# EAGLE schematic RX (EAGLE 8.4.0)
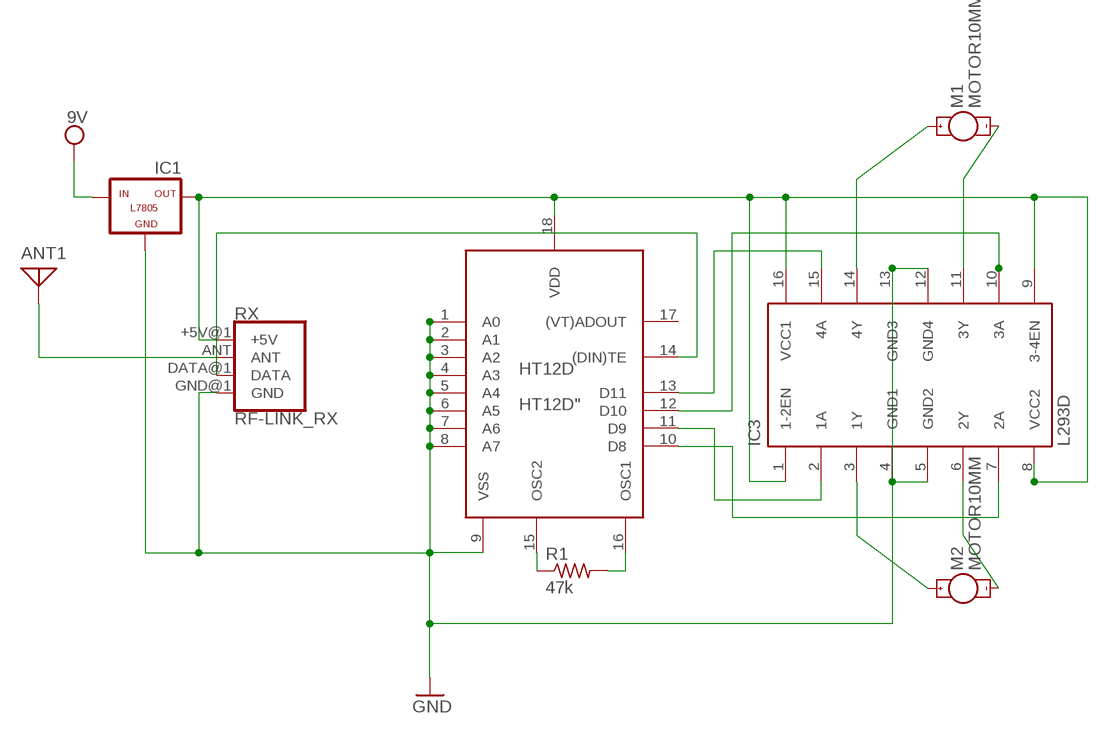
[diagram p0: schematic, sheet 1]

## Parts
ANT1  ANTENNA  [PAD-01]
HT12D  HT12D"  [18-DIP-A]
IC1  5V  L7805  [78XXL]
IC3  L293D  [DIL16]
M1  MOTOR10MM  [VIBE-MOTOR-10MM]
M2  MOTOR10MM  [VIBE-MOTOR-10MM]
R1  47k  R-US_R0201  [R0201]
RX  RF-LINK_RX  [RF-LINK_RX]

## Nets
GND: HT12D.1(A0) HT12D.2(A1) HT12D.3(A2) HT12D.4(A3) HT12D.5(A4) HT12D.6(A5) HT12D.7(A6) HT12D.8(A7) HT12D.9(VSS) IC1.GND IC3.4(GND1) IC3.5(GND2) IC3.12(GND4) IC3.13(GND3) RX.GND@1(GND)
N$1: IC3.6(2Y) M2.-
N$2: ANT1.1 RX.ANT
N$3: HT12D.12(D10) IC3.10(3A)
N$4: IC3.11(3Y) M1.-
N$5: HT12D.15(OSC2) R1.1
N$6: HT12D.16(OSC1) R1.2
N$7: HT12D.14((DIN)TE) RX.DATA@1(DATA)
N$9: HT12D.18(VDD) IC1.OUT IC3.1(1-2EN) IC3.8(VCC2) IC3.9(3-4EN) IC3.16(VCC1) RX.+5V@1(+5V)
N$11: HT12D.10(D8) IC3.7(2A)
N$12: HT12D.11(D9) IC3.2(1A)
N$13: IC3.14(4Y) M1.+
N$14: HT12D.13(D11) IC3.15(4A)
N$15: IC3.3(1Y) M2.+
VSS: IC1.IN ; supply symbol labelled 9V
Unconnected: HT12D.17((VT)ADOUT)

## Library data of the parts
ANT1 = discrete:ANTENNA: Antenna
HT12D = holtek:HT12D: decoder = receiver ic
IC1 = l7805:L7805: VOLTAGE REGULATOR
IC3 = st-microelectronics:L293D: PUSH-PULL 4 CHANNEL DRIVER; MPN: L293D; OC_FARNELL: 9589619; OC_NEWARK: 56P8249
M1 M2 = SparkFun-Electromechanical:MOTOR: Motor (Single-Phase); PROD_ID: COMP-08572; SF_SKU: ROB-08449
R1 = rcl:R-US_: RESISTOR, American symbol
RX = SparkFun-RF:RF-LINK_RX: RF Link Receiver (434 MHz, 315 MHz) These wireless receivers work with equivalent transmitters. They can easily fit into a breadboard and work well with microcontrollers to create a very simple wireless data link. Since these are only receivers, they will only work communicating data one-way, you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; SF_ID: WRL-10533

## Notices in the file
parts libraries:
SparkFun-RF: Licensing: Creative Commons ShareAlike 4.0 International - https://creativecommons.org/licenses/by-sa/4.0
